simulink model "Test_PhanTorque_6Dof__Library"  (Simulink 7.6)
settings: Solver=ode3  StartTime=0.0  StopTime=inf  RelTol=1e-3
libraries: PhanTorque_6Dof_Library_64Bits x6

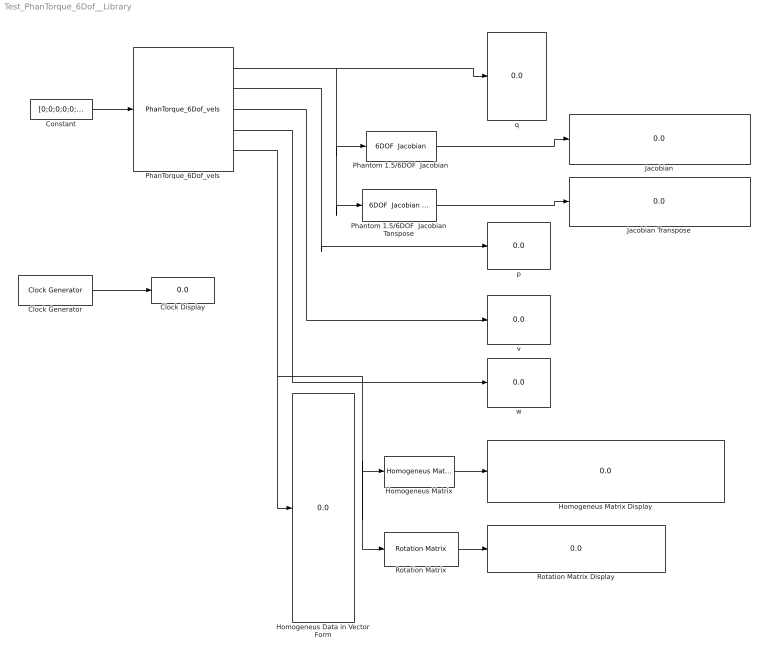
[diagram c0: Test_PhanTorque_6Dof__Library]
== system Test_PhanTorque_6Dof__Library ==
  Clock Display : Display
  Clock Generator : PhanTorque_6Dof_Library_64Bits/Clock Generator
  Constant : Constant  Value=[0;0;0;0;0;0]
  Homogeneus Data in Vector Form : Display
  Homogeneus Matrix : PhanTorque_6Dof_Library_64Bits/Homogeneus Matrix  SystemSampleTime=-1
  Homogeneus Matrix Display : Display
  Jacobian : Display
  Jacobian Transpose : Display
  PhanTorque_6Dof_vels : PhanTorque_6Dof_Library_64Bits/PhanTorque_6Dof_vels  Haptic_Name='Default PHANToM'  kd=0
  Phantom 1.5/6DOF  Jacobian : PhanTorque_6Dof_Library_64Bits/Phantom 1.5//6DOF  Jacobian  SystemSampleTime=-1
  Phantom 1.5/6DOF  Jacobian Tanspose : PhanTorque_6Dof_Library_64Bits/Phantom 1.5//6DOF  Jacobian Tanspose  SystemSampleTime=-1
  Rotation Matrix : PhanTorque_6Dof_Library_64Bits/Rotation Matrix  SystemSampleTime=-1
  Rotation Matrix Display : Display
  p : Display
  q : Display
  v : Display
  w : Display
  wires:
  PhanTorque_6Dof_vels/5 -> Homogeneus Data in Vector Form/1, Homogeneus Matrix/1, Rotation Matrix/1
  PhanTorque_6Dof_vels/2 -> p/1
  PhanTorque_6Dof_vels/1 -> q/1, Phantom 1.5/6DOF  Jacobian/1, Phantom 1.5/6DOF  Jacobian Tanspose/1
  Phantom 1.5/6DOF  Jacobian/1 -> Jacobian/1
  Rotation Matrix/1 -> Rotation Matrix Display/1
  Homogeneus Matrix/1 -> Homogeneus Matrix Display/1
  Clock Generator/1 -> Clock Display/1
  Phantom 1.5/6DOF  Jacobian Tanspose/1 -> Jacobian Transpose/1
  PhanTorque_6Dof_vels/3 -> v/1
  Constant/1 -> PhanTorque_6Dof_vels/1
  PhanTorque_6Dof_vels/4 -> w/1
